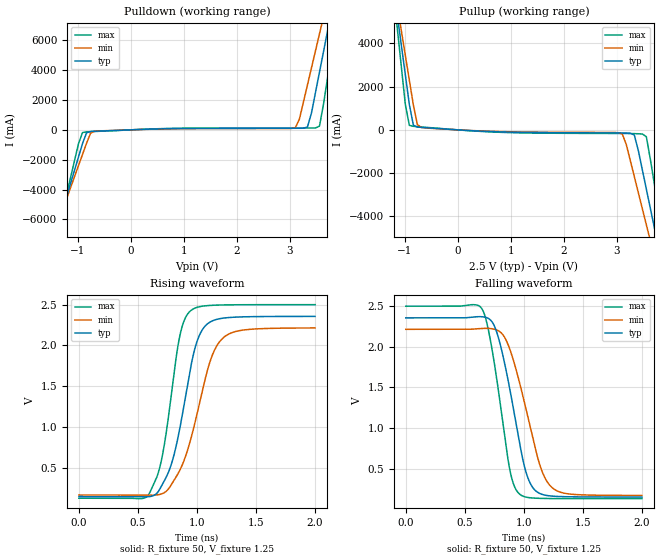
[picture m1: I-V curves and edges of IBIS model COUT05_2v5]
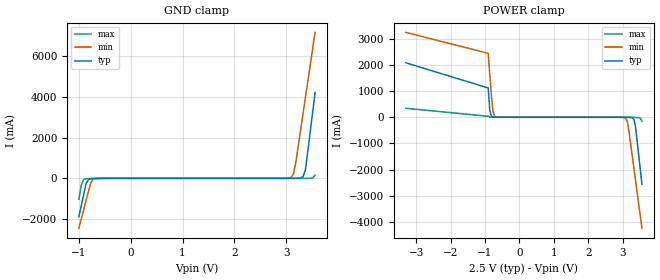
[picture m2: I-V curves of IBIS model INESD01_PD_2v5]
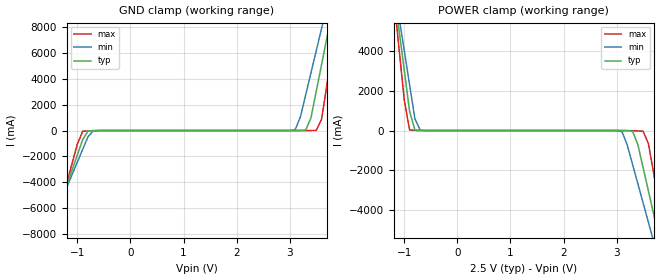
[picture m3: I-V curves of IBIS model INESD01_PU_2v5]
|   This file is an IBIS representation of the   |
|   Integrated Device Technology, Inc.   |
|   ICS8344I   |
|   LOW SKEW, 1-TO-24 DIFFERENTIAL-TO-LVCMOS/LVTTL FANOUT BUFFER   |
[IBIS Ver]   4.1
[File name]   8344i.ibs
[File Rev]   1.0
[Date]   9 Jun 2009 | Last modified
|   Sep 07 2007 | Generated
[Source]   Originated at Integrated Devices Technology, Inc.
[Disclaimer]
IDT hereby grants the user of this IBIS model a non-exclusive,
nontransferable license to use this IBIS model under the following terms.
Before using this IBIS model, the user should read this license.
If the user does not accept these terms,  the IBIS model should be
returned to IDT within 30 days.
   The user is granted this license only to use the IBIS model and
is not granted rights to sell, load, rent, lease or license the IBIS
model in whole or in part, or in modified form to anyone other than
user. User may modify the IBIS model to suit its specific
applications but rights to derivative works and such modifications
shall belong to IDT.
   This IBIS model is provided on an "AS IS" basis and IDT makes
absolutely no warranty with respect to the information contained
herein. IDT DISCLAIMS AND CUSTOMER WAIVES ALL WARRANTIES, EXPRESS
OR IMPLIED, INCLUDING WARRANTIES OF MERCHANTABILITY OR FITNESS FOR
A PARTICULAR PURPOSE. The entire risk as to quality and performance
is with the Customer. ACCORDINGLY, IN NO EVENT SHALL THE COMPANY BE
LIABLE FOR ANY DAMAGES, WHETHER IN CONTRACT OR TORT,INCLUDING ANY
LOST PROFITS OR OTHER INCIDENTAL, CONSEQUENTIAL, EXEMPLARY, OR
PUNITIVE DAMAGES ARISING OUT OF THE USE OR APPLICATION OF THE IBIS
model provided in this package. Further, IDT reserves the right to
make changes without notice to any product herein to improve
reliability, function, or design. IDT does not convey any license
under patent rights or any other intellectual property rights,
including those of third parties.
   IDT is not obligated to provide maintenance or support
for the licensed IBIS model.
[Copyright]   Copyright 2007 by Integrated Device Technology, Inc.
[Component]   ICS8344IY
[Manufacturer] Integrated Devices Technology, Inc.
[Package]
|LQFP48
|lead + wire   typ   min   max
R_pkg   220.4m   212.5m   238m
L_pkg   1.841nH   1.708nH   1.974n
C_pkg   0.316pF   0.2907pF   0.338pF
[Pin] signal_name   model_name   R_pin   L_pin   C_pin
1   Q16   COUT05   238m   1.974n   0.338p
2   Q17   COUT05   225m   1.831n   0.330p
3   VDDO   POWER   220m   1.781n   0.323p
4   GND   GND   214m   1.732n   0.312p
5   Q18   COUT05   214m   1.709n   0.305p
6   Q19   COUT05   213m   1.708n   0.291p
7   Q20   COUT05   213m   1.708n   0.291p
8   Q21   COUT05   214m   1.709n   0.305p
9   VDDO   POWER   214m   1.732n   0.312p
10  GND   GND   220m   1.781n   0.323p
11  Q22   COUT05   225m   1.831n   0.330p
12  Q23   COUT05   238m   1.974n   0.338p
13  CLK_SEL   INESD01_PD   238m   1.974n   0.338p
14  GND   GND   225m   1.831n   0.330p
15  VDD   POWER   220m   1.781n   0.323p
16  nCLK1   INESD01_PU   214m   1.732n   0.312p
17  CLK1   INESD01_PD   214m   1.709n   0.305p
18  GND   GND   213m   1.708n   0.291p
19  VDD   POWER   213m   1.708n   0.291p
20  nCLK0   INESD01_PU   214m   1.709n   0.305p
21  CLK0   INESD01_PD   214m   1.732n   0.312p
22  OE3   INESD01_PU   220m   1.781n   0.323p
23  OE2   INESD01_PU   225m   1.831n   0.330p
24  OE1   INESD01_PU   238m   1.974n   0.338p
25  Q0   COUT05   238m   1.974n   0.338p
26  Q1   COUT05   225m   1.831n   0.330p
27  GND   GND   220m   1.781n   0.323p
28  VDDO   GND   214m   1.732n   0.312p
29  Q2   COUT05   214m   1.709n   0.305p
30  Q3   COUT05   213m   1.708n   0.291p
31  Q4   COUT05   213m   1.708n   0.291p
32  Q5   COUT05   214m   1.709n   0.305p
33  GND   GND   214m   1.732n   0.312p
34  VDDO   POWER   220m   1.781n   0.323p
35  Q6   COUT05   225m   1.831n   0.330p
36  Q7   COUT05   238m   1.974n   0.338p
37  Q8   COUT05   238m   1.974n   0.338p
38  Q9   COUT05   225m   1.831n   0.330p
39  VDDO   POWER   220m   1.781n   0.323p
40  GND   GND   214m   1.732n   0.312p
41  Q10   COUT05   214m   1.709n   0.305p
42  Q11   COUT05   213m   1.708n   0.291p
43  Q12   COUT05   213m   1.708n   0.291p
44  Q13   COUT05   214m   1.709n   0.305p
45  VDDO   POWER   214m   1.732n   0.312p
46  GND   GND   220m   1.781n   0.323p
47  Q14   COUT05   225m   1.831n   0.330p
48  Q15   COUT05   238m   1.974n   0.338p
[Diff Pin]  inv_pin  vdiff tdelay_typ tdelay_min  tdelay_max
21   20   NA   0  0  0
17   16   NA   0  0  0
[Model Selector] COUT05
COUT05_2v5  Buffer selection for 2v5
COUT05_3v3  Buffer selection for 3v3
[Model Selector] INESD01_PD
INESD01_PD_2v5  Buffer selection for 2v5
INESD01_PD_3v3  Buffer selection for 3v3
[Model Selector] INESD01_PU
INESD01_PU_2v5  Buffer selection for 2v5
INESD01_PU_3v3  Buffer selection for 3v3
| Models and submodels in the file (6): COUT05_2v5 (Output), INESD01_PD_2v5 (Input), INESD01_PU_2v5 (Input), COUT05_3v3 (Output), INESD01_PD_3v3 (Input), INESD01_PU_3v3 (Input)
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[Model] COUT05_2v5
Model_type   Output
Polarity   Non-Inverting
|   typ   min   max
C_comp   2pF   1.5pF   2.5pF
Vmeas = 1.25V
Rref = 50
Cref = 50
Vref = 1.25V
|   typ   min   max
[Voltage range]   2.5V   2.375V   2.625V
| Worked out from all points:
|   slope of the pulldown table from 0 to 0.375 V, typ, clamps not added: 7.84 ohm
|   slope of the pullup table from 0 to 0.375 V, typ, clamps not added: 7.17 ohm
|   rising waveform, R_fixture 50, V_fixture 1.25: 20-80 % time 181ps typ, 224ps min, 142ps max; typ from 0.154 V to 2.35 V
|   falling waveform, R_fixture 50, V_fixture 1.25: 20-80 % time 175ps typ, 211ps min, 143ps max; typ from 2.35 V to 0.154 V
[Pulldown]
|Voltage   I (typ)   I (min)   I (max)
-2.5V     -19.75A    -17.35A    -23.82A
-1.439V   -7.206A    -6.887A    -7.808A
-1.364V   -6.308A    -6.139A    -6.662A
-909.1mV  -921.7mA   -1.65A     -183.6mA
-833.3mV  -199.2mA   -901.6mA   -138mA
-681.8mV  -95.6mA    -94.51mA   -111.1mA
3.106V    103.9mA    147.7mA    121.5mA
3.333V    187.7mA    3.001A     122.2mA
3.561V    3.866A     6.429A     248.4mA
3.712V    6.611A     8.717A     3.472A
3.864V    9.357A     11A        6.981A
5V        29.99A     28.19A     33.35A
[Pullup]
|Voltage   I (typ)   I (min)   I (max)
-2.5V     30.11A     26.42A     36.38A
-1.136V   5.3A       5.738A     4.69A
-1.061V   3.921A     4.589A     2.928A
-909.1mV  1.162A     2.291A     208.3mA
-681.8mV  112.8mA    108.8mA    133.2mA
3.106V    -144.5mA   -188.3mA   -168.5mA
3.333V    -240.4mA   -2.164A    -175.3mA
3.485V    -1.852A    -3.654A    -191.8mA
3.561V    -2.745A    -4.399A    -320.2mA
3.712V    -4.534A    -5.89A     -2.513A
3.864V    -6.324A    -7.381A    -4.797A
5V        -19.75A    -18.57A    -21.94A
[Ramp]
|   typ   min   max
dV/dt_r   1.763/0.291n   1.634/0.358n   1.895/0.227n
dV/dt_f   1.772/0.26n   1.642/0.314n   1.906/0.211n
R_load =   50.0000
[Rising Waveform]
R_fixture = 50
V_fixture = 1.25   |Vcc_typ
V_fixture_min = 1.1875 |Vcc_min
V_fixture_max = 1.3125 |Vcc_max
C_fixture = 0.0p
| Time   typ   min   max
0s        154.1mV    173.3mV    133.8mV
594.6ps   153.1mV    171mV      187.8mV
694.7ps   270mV      184.1mV    568.7mV
782.8ps   548.4mV    298.9mV    1.397V
860.9ps   1.034V     493.9mV    2.157V
948.9ps   1.748V     863.7mV    2.427V
1.049ns   2.2V       1.466V     2.48V
1.131ns   2.301V     1.885V     2.49V
1.223ns   2.334V     2.094V     2.495V
2ns       2.355V     2.214V     2.498V
[Falling Waveform]
R_fixture = 50
V_fixture = 1.25   |Vcc_typ
V_fixture_min = 1.1875 |Vcc_min
V_fixture_max = 1.3125 |Vcc_max
C_fixture = 0.0p
| Time   typ   min   max
0s        2.355V     2.214V     2.498V
646.6ps   2.368V     2.225V     2.462V
702.7ps   2.345V     2.225V     2.186V
780.8ps   2.131V     2.199V     1.501V
882.9ps   1.467V     1.963V     477.1mV
965ps     809.8mV    1.551V     188.8mV
1.065ns   293.1mV    943.2mV    143.1mV
1.149ns   189.4mV    489.6mV    137.3mV
1.235ns   165.9mV    275.2mV    135.3mV
2ns       154.1mV    173.6mV    133.8mV
[Model] INESD01_PD_2v5
Model_type   Input
Polarity   Non-Inverting
Vinl = 0.8V
Vinh = 2.0V
|   typ   min   max
C_comp   2pF   1.5pF   2.5pF
|   typ   min   max
[Voltage range]  2.5V   2.375V   2.625V
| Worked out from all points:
|   GND clamp passes 1 mA (typ) near -0.55 V on its own axis
|   POWER clamp passes 1 mA (typ) near -0.68 V on its own axis
[GND_clamp]
|Voltage I(typ)   I(min)   I(max)
-1V       -1.886A    -2.451A    -1.028A
-953.5mV  -1.338A    -1.994A    -328mA
-907mV    -789.6mA   -1.537A    -53.04mA
-860.5mV  -251.4mA   -1.081A    -21.51mA
-767.5mV  -17.28mA   -198.8mA   -10.01mA
-674.5mV  -5.28mA    -15.38mA   -3.684mA
3.092V    224.5uA    49.06mA    51.52uA
3.139V    500.8uA    208.3mA    52.98uA
3.185V    1.252mA    774.6mA    56.66uA
3.325V    81.55mA    3.177A     200uA
3.371V    416.9mA    3.978A     464.6uA
3.557V    4.225A     7.185A     159.2mA
[POWER_clamp]
|Voltage   I(typ)   I(min)   I(max)
-3.3V     2.083A     3.246A     343.1mA
-907mV    1.122A     2.445A     37.78mA
-860.5mV  267.5mA    1.644A     5.973mA
-814mV    47.03mA    844mA      1.727mA
-767.5mV  9.66mA     215.3mA    677uA
-674.5mV  960.6uA    12.66mA    131.4uA
3.092V    -1.849mA   -49.09mA   -51.51uA
3.139V    -3.491mA   -186mA     -159.7uA
3.325V    -84.03mA   -1.955A    -5.102mA
3.371V    -365.4mA   -2.411A    -8.31mA
3.51V     -2.01A     -3.782A    -35.44mA
3.557V    -2.558A    -4.239A    -152.3mA
[Model] INESD01_PU_2v5
Model_type   Input
Polarity   Non-Inverting
Vinl = 1.4V
Vinh = 1.85V
|   typ   min   max
C_comp   2pF   1.5pF   2.5pF
|   typ   min   max
[Voltage range]  2.5V   2.375V   2.625V
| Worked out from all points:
|   GND clamp passes 1 mA (typ) near -0.54 V on its own axis
|   POWER clamp passes 1 mA (typ) near -0.66 V on its own axis
[GND_clamp]
|Voltage   I(typ)   I(min)   I(max)
-2.5V     -19.6A     -17.18A    -23.67A
-1.6V     -8.969A    -8.332A    -10.1A
-1.5V     -7.788A    -7.349A    -8.588A
-900mV    -707.1mA   -1.46A     -57.43mA
-700mV    -7.027mA   -24.05mA   -13.28mA
3.1V      199.2uA    53.94mA    11.78uA
3.3V      28.4mA     2.748A     652.4uA
3.5V      3.045A     6.192A     15.72mA
3.6V      5.115A     7.914A     872.4mA
3.7V      7.185A     9.638A     3.52A
3.9V      11.33A     13.09A     8.818A
5V        34.14A     32.07A     37.99A
[POWER_clamp]
|Voltage   I(typ)   I(min)   I(max)
-1.5V     9.257A     9.207A     9.48A
-1.2V     7.185A     7.484A     6.83A
-1.1V     5.115A     5.761A     4.182A
-900mV    976.9mA    2.318A     34.23mA
-700mV    1.582mA    24.31mA    1.044mA
3.1V      -2.107mA   -51.03mA   -534.5uA
3.3V      -35.62mA   -1.705A    -10.86mA
3.5V      -1.886A    -3.666A    -39.41mA
3.6V      -3.066A    -4.647A    -666.9mA
3.8V      -5.426A    -6.612A    -3.684A
3.9V      -6.607A    -7.595A    -5.193A
5V        -19.6A     -18.41A    -21.79A
